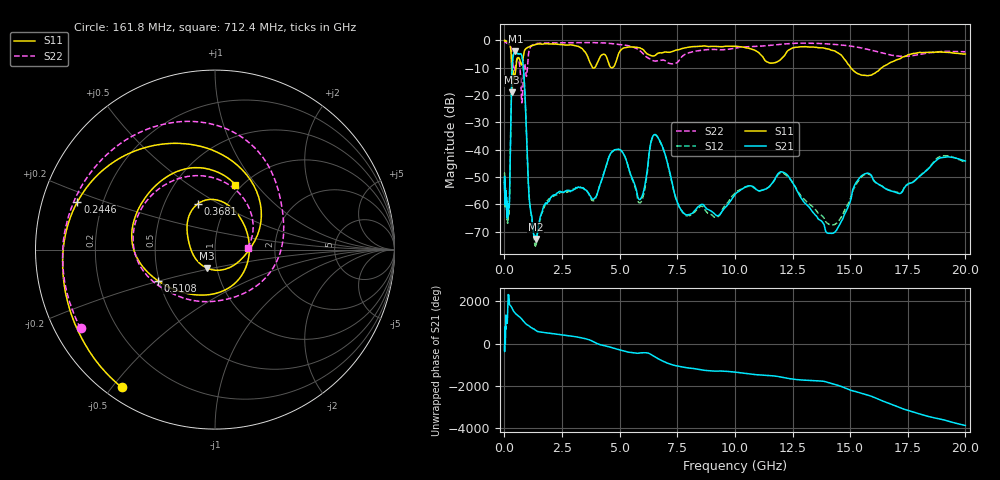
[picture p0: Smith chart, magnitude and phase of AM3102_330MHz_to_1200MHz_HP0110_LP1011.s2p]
! Date/Time: Tue, Sep 11, 2018 5:15 PM
! Network Analyzer: Agilent Technologies E8362B Rev: A.07.50.63
! Sweep from 0.010 to 20.000 GHz, 1601 Points, Sweep Type: LOG
! Power Supply: 4.949 V, 0.001 A
# Hz S DB R 50
!freq MagS11 AngS11 MagS21 AngS21 MagS12 AngS12 MagS22 AngS22
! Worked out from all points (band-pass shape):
!   1601 points, 10 MHz to 20 GHz, reference 50 ohm
!   highest |S21| = -3.97 dB at 475.7 MHz (marker M1); lowest = -72.6 dB at 1.359 GHz (marker M2)
!   |S21| within 3 dB of the highest: 359.6 MHz to 789.4 MHz (429.9 MHz wide, 74.8 % of centre)
!   lowest |S11| = -19.0 dB at 337.9 MHz (marker M3), VSWR 1.25, Z = 44.7 - j9.3 ohm
!   |S11| at or under -10 dB: 314.9 MHz to 497.4 MHz (182.6 MHz wide, 44.9 % of centre); 3.831 GHz to 3.912 GHz (80.52 MHz wide, 2.08 % of centre); 15.03 GHz to 16.37 GHz (1.343 GHz wide, 8.56 % of centre)
!   |S22| runs from -22.8 to -0.3 dB; largest |S21 - S12| = 0.011
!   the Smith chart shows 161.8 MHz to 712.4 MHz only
!   S11 on the Smith chart (normalised r, x): 161.8 MHz: 0.05, -0.53; 244.6 MHz: 0.11, +0.17; 368.1 MHz: 0.73, +0.40; 510.8 MHz: 0.49, -0.19; 712.4 MHz: 0.94, +0.78
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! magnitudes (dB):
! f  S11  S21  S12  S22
! 10 MHz  0.0  -51.2  -48.5  -0.3
! 35.55 MHz  0.0  -57.1  -56.0  -0.5
! 126.4 MHz  -0.4  -63.9  -61.6  -1.1
! 161.8 MHz  -0.7  -63.1  -63.2  -1.2
! 244.6 MHz  -1.8  -47.6  -47.6  -1.8
! 337.9 MHz  -19.0  -9.5  -9.6  -6.3
! 368.1 MHz  -11.3  -6.4  -6.5  -8.5
! 447.2 MHz  -13.5  -4.1  -4.1  -10.4
! 475.7 MHz  -11.8  -4.0  -4.0  -9.5
! 510.8 MHz  -8.8  -4.2  -4.3  -8.0
! 712.4 MHz  -8.5  -4.9  -4.9  -14.8
! 841.2 MHz  -4.8  -11.8  -11.9  -10.5
! 1.359 GHz  -1.5  -72.6  -74.2  -1.2
! 1.59 GHz  -1.3  -63.9  -64.1  -1.0
! 3.884 GHz  -10.1  -58.0  -58.6  -0.8
! 4.855 GHz  -7.5  -39.9  -39.9  -1.3
! 5.652 GHz  -2.4  -52.7  -53.3  -2.6
! 6.612 GHz  -4.9  -34.9  -34.9  -7.5
! 7.845 GHz  -2.7  -63.6  -63.9  -5.0
! 12.09 GHz  -6.1  -48.2  -48.6  -1.3
! 14.14 GHz  -3.4  -70.6  -67.5  -1.3
! 20 GHz  -5.0  -44.1  -44.7  -4.1
